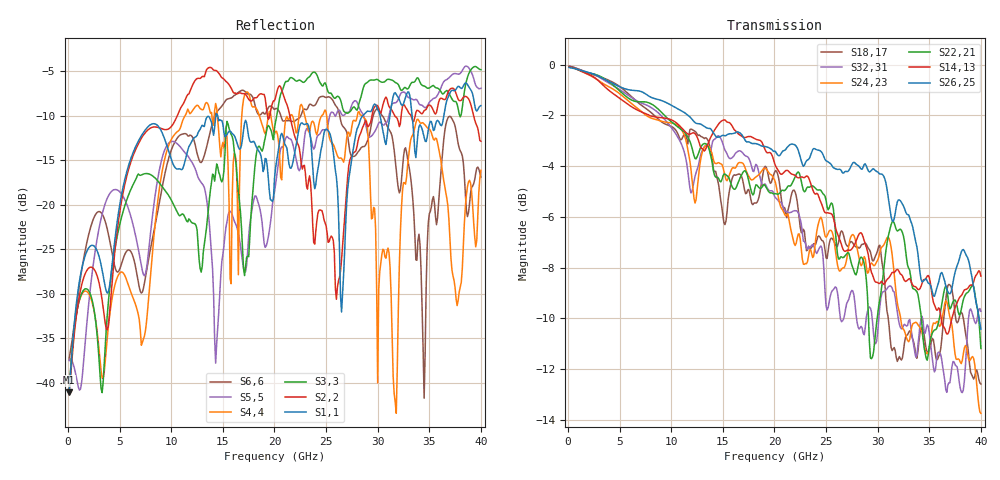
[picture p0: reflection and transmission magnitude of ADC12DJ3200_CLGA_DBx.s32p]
! Touchstone file
! Texas Instruments 4/21/2021
! ADC12DJ3200QML-SP
! Package-type  CLGA [BGA]
! pins/pkg drawing  196-pin ZMX
! CLGA Ceramic Package without columns (ceramic land grid array)
! High-speed serialized data output for channel B, lane 0-7
# GHZ S MA R 50.000000
! Port[1] = DB0N_BGA_J14
! Port[2] = DB0N_DIE_6
! Port[3] = DB0P_BGA_K14
! Port[4] = DB0P_DIE_5
! Port[5] = DB1N_BGA_L14
! Port[6] = DB1N_DIE_8
! Port[7] = DB1P_BGA_M14
! Port[8] = DB1P_DIE_7
! Port[9] = DB2N_BGA_P13
! Port[10] = DB2N_DIE_10
! Port[11] = DB2P_BGA_P12
! Port[12] = DB2P_DIE_9
! Port[13] = DB3N_BGA_P11
! Port[14] = DB3N_DIE_12
! Port[15] = DB3P_BGA_P10
! Port[16] = DB3P_DIE_11
! Port[17] = DB4N_BGA_J13
! Port[18] = DB4N_DIE_14
! Port[19] = DB4P_BGA_K13
! Port[20] = DB4P_DIE_13
! Port[21] = DB5N_BGA_L13
! Port[22] = DB5N_DIE_16
! Port[23] = DB5P_BGA_M13
! Port[24] = DB5P_DIE_15
! Port[25] = DB6N_BGA_N13
! Port[26] = DB6N_DIE_18
! Port[27] = DB6P_BGA_N12
! Port[28] = DB6P_DIE_17
! Port[29] = DB7N_BGA_N11
! Port[30] = DB7N_DIE_20
! Port[31] = DB7P_BGA_N10
! Port[32] = DB7P_DIE_19
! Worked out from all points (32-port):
!   400 points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, 100 MHz to 40 GHz, reference 50 ohm
!   strongest paths, dB at 100 MHz, 10.1 GHz, 20.1 GHz, 30.1 GHz, 40 GHz:
!     S26,25: -0.1, -1.6, -3.4, -4.3, -10.4
!     S14,13: -0.1, -2.2, -4.0, -8.6, -8.3
!     S22,21: -0.1, -2.3, -5.1, -9.5, -11.2
!     S24,23: -0.1, -2.3, -4.7, -7.6, -13.7
!     S32,31: -0.1, -2.5, -5.3, -10.0, -9.7
!     S18,17: -0.1, -2.5, -4.2, -7.2, -12.6
!   lowest |S11| = -41.1 dB at 100 MHz (marker M1), VSWR 1.02, Z = 50.8 - j0.278 ohm
!   |S11| at or under -10 dB: start of sweep to 14.34 GHz; 14.5 GHz to 28.56 GHz (14.06 GHz wide, 65.3 % of centre); 33.34 GHz to 36.41 GHz (3.074 GHz wide, 8.82 % of centre)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
